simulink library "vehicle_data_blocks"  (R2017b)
settings: Solver=ode1  StartTime=0.0  StopTime=Inf  FixedStep=0.001  RelTol=1e-3  EnableMultiTasking=on
PostLoadFcn:
  | , if any(exist('dsrtsu_mdlpostloadfcn', 'file') == [2, 3, 6]), try dsrtsu_mdlpostloadfcn('Execute', bdroot); catch fprintf('Error in PostLoadFcn (dsrtsu_mdlpostloadfcn) for model "%s":\n %s\n', bdroot, lasterr); end, end,
libraries: rtican x11

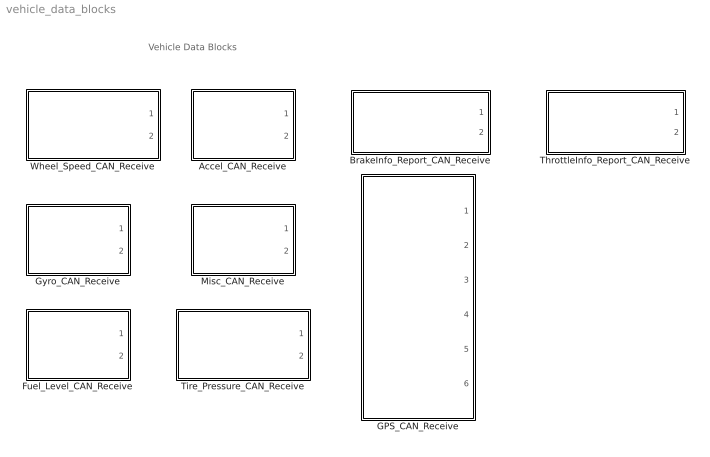
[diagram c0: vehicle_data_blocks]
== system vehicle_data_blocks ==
  note: Vehicle Data Blocks
  Accel_CAN_Receive : Subsystem
  BrakeInfo_Report_CAN_Receive : Subsystem
  Fuel_Level_CAN_Receive : Subsystem
  GPS_CAN_Receive : Subsystem
  Gyro_CAN_Receive : Subsystem
  Misc_CAN_Receive : Subsystem
  ThrottleInfo_Report_CAN_Receive : Subsystem
  Tire_Pressure_CAN_Receive : Subsystem
  Wheel_Speed_CAN_Receive : Subsystem

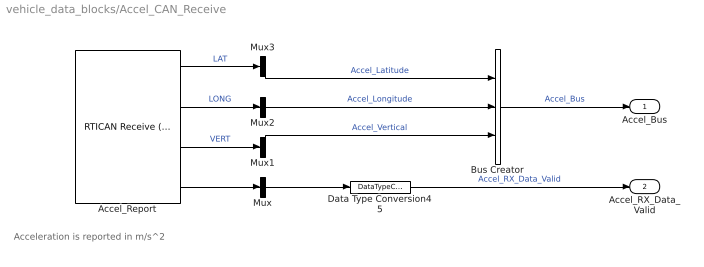
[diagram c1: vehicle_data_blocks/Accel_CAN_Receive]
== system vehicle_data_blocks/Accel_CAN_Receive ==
  note: Acceleration is reported in m/s^2
  Accel_Report : rtican/RTICAN Receive (RX)   Reserved1=[]  Reserved2=[]  Reserved3=[]  Reserved4=[]  SfcnMessage=[]  Msg_Struct=[]  BoardTypeNo=[]  BoardNo=[]  ChannelNo=[]  Parameters=[]  DialogFcn=[]  UnitName=[]  Revision=[]  UnitValues=[]  DSProperties=struct('RTI',struct('Version',uint32(5),'BlockType',struct('isSLSource',uint8(1),'isSLSink',uint8(1),'isHWSource',uint8(0),'isHWSink',uint8(0),'isSetup',uint8(0),'isInline',uint8(1),'isNonInline',uint8(0),'isInterrupt',uint8(0),'isChannelwise',uint8(0)),'IOBoardType','RTICAN','UnitType','MESSAGE','Identifier','RX','DialogType','MSVC','BlockSet','RTICAN','SlaveProcessor','CAN'))  RTIBlockInterface=struct('OutputPortsWidth',int32([1 1 1 1]),'OutputPortsActive',[1 1 1 1],'OutputPortsName',{{'LAT','LONG','VERT',['RX status']}},'OutputPortsDataType',{{'SS_DOUBLE','SS_DOUBLE','SS_DOUBLE','SS_DOUBLE'}},'OutputPortsLabel',{{'LAT','LONG','VERT',''}},'OutputPortsLabelMode','ON','InputPortsWidth',int32(0),'InputPortsActive',0,'DialogFcn','rtican_message_interface_gui','BlockDisplay',{{'','center'}},'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  RTIBlockParameters=struct('BoardTypeNo',{{1,'OFF',[]}},'BoardNo',{{1,'ON',[1 16]}},'ChannelNo',{{1,'ON',[1 2]}},'Parameters',{{struct('DataFileSupport',struct('DataFileSelectedMaster',1,'DataFileSelectedLocal',1,'DataFileName','c:\repos\forddrivebywire\dataspeedbywire.dbc|','DataFileDate',['06-Sep-2016 16:47:06'],'SelectedFile','dataspeedbywire_20160909.dbc','InterfaceFcn','rtican_dbc_file_parser'),'Options',struct(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  RTISFcnParameters=struct('SFcnRTICANMessage','struct','TLCFileName','char')  RTIBlockParaDefault=struct('BoardTypeNo',4302,'BoardNo',1,'ChannelNo',1,'Parameters',struct('DataFileSupport',struct('DataFileSelectedMaster',0,'DataFileSelectedLocal',0,'DataFileName','','DataFileDate','','SelectedFile',['<no file selected>']),'Options',struct('StatusSelected',1,'TimeSelected',1,'DeltaTimeSelected',1,'BytePortSelected',0,'MessageLengthSelected',0,'TriggerPort',struct('Selected',0,'TriggerType','risi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
  Bus Creator : BusCreator  Inputs=3
  Data Type Conversion45 : DataTypeConversion  OutDataTypeStr=boolean
  Mux{,1..3} (4 alike) : Mux  Inputs=1
  Accel_Bus : Outport
  Accel_RX_Data_Valid : Outport  Port=2
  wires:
  Data Type Conversion45/1 -> Accel_RX_Data_Valid/1  "Accel_RX_Data_Valid"
  Mux1/1 -> Bus Creator/3  "Accel_Vertical"
  Mux2/1 -> Bus Creator/2  "Accel_Longitude"
  Mux3/1 -> Bus Creator/1  "Accel_Latitude"
  Mux/1 -> Data Type Conversion45/1
  Accel_Report/4 -> Mux/1
  Accel_Report/3 -> Mux1/1  "VERT"
  Accel_Report/2 -> Mux2/1  "LONG"
  Accel_Report/1 -> Mux3/1  "LAT"
  Bus Creator/1 -> Accel_Bus/1  "Accel_Bus"

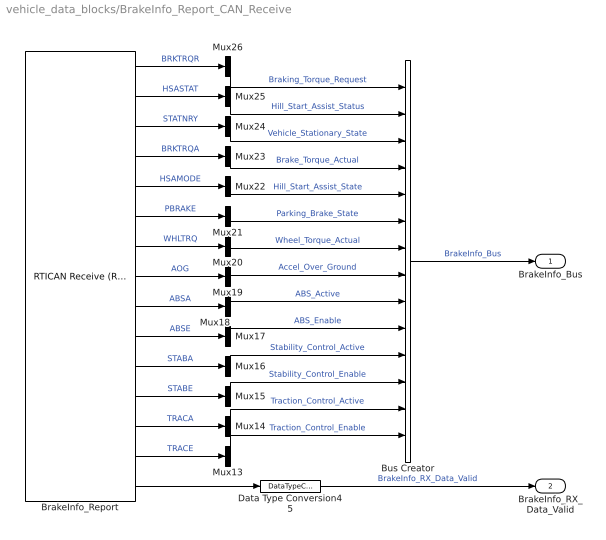
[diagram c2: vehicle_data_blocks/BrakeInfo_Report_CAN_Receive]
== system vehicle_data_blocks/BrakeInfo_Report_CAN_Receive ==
  BrakeInfo_Report : rtican/RTICAN Receive (RX)   Reserved1=[]  Reserved2=[]  Reserved3=[]  Reserved4=[]  SfcnMessage=[]  Msg_Struct=[]  BoardTypeNo=[]  BoardNo=[]  ChannelNo=[]  Parameters=[]  DialogFcn=[]  UnitName=[]  Revision=[]  UnitValues=[]  DSProperties=struct('RTI',struct('Version',uint32(5),'BlockType',struct('isSLSource',uint8(1),'isSLSink',uint8(1),'isHWSource',uint8(0),'isHWSink',uint8(0),'isSetup',uint8(0),'isInline',uint8(1),'isNonInline',uint8(0),'isInterrupt',uint8(0),'isChannelwise',uint8(0)),'IOBoardType','RTICAN','UnitType','MESSAGE','Identifier','RX','DialogType','MSVC','BlockSet','RTICAN','SlaveProcessor','CAN'))  RTIBlockInterface=struct('OutputPortsWidth',int32([1 1 1 1 1 1 1 1 1 1 1 1 1 1 1]),'OutputPortsActive',ones(1,15),'OutputPortsName',{{'BRKTRQR','HSASTAT','STATNRY','BRKTRQA','HSAMODE','PBRAKE','WHLTRQ','AOG','ABSA','ABSE','STABA','STABE','TRACA','TRACE',['RX status']}},'OutputPortsDataType',{{'SS_UINT16','SS_UINT8','SS_BOOLEAN','SS_UINT16','SS_UINT8','SS_UINT8','SS_INT16','SS_DOUBLE','SS_BOOLEAN','SS_BOOLEAN','SS_B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  RTIBlockParameters=struct('BoardTypeNo',{{1,'OFF',[]}},'BoardNo',{{1,'ON',[1 16]}},'ChannelNo',{{1,'ON',[1 2]}},'Parameters',{{struct('DataFileSupport',struct('DataFileSelectedMaster',1,'DataFileSelectedLocal',1,'DataFileName','c:\users\jsmith.dsi\documents\projects\forddrivebywire\dspace\lib\dataspeedbywire.dbc|','DataFileDate',['06-Sep-2016 16:47:06'],'SelectedFile','dataspeedbywire.dbc','InterfaceFcn','rtican_dbc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  RTISFcnParameters=struct('SFcnRTICANMessage','struct','TLCFileName','char')  RTIBlockParaDefault=struct('BoardTypeNo',4302,'BoardNo',1,'ChannelNo',1,'Parameters',struct('DataFileSupport',struct('DataFileSelectedMaster',0,'DataFileSelectedLocal',0,'DataFileName','','DataFileDate','','SelectedFile',['<no file selected>']),'Options',struct('StatusSelected',1,'TimeSelected',1,'DeltaTimeSelected',1,'BytePortSelected',0,'MessageLengthSelected',0,'TriggerPort',struct('Selected',0,'TriggerType','risi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
  Bus Creator : BusCreator  Inputs=14
  Data Type Conversion45 : DataTypeConversion  OutDataTypeStr=boolean
  Mux{13..26} (14 alike) : Mux  Inputs=1
  BrakeInfo_Bus : Outport
  BrakeInfo_RX_Data_Valid : Outport  Port=2
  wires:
  BrakeInfo_Report/15 -> Data Type Conversion45/1
  Data Type Conversion45/1 -> BrakeInfo_RX_Data_Valid/1  "BrakeInfo_RX_Data_Valid"
  BrakeInfo_Report/14 -> Mux13/1  "TRACE"
  BrakeInfo_Report/13 -> Mux14/1  "TRACA"
  BrakeInfo_Report/1 -> Mux26/1  "BRKTRQR"
  BrakeInfo_Report/2 -> Mux25/1  "HSASTAT"
  BrakeInfo_Report/3 -> Mux24/1  "STATNRY"
  BrakeInfo_Report/4 -> Mux23/1  "BRKTRQA"
  BrakeInfo_Report/5 -> Mux22/1  "HSAMODE"
  BrakeInfo_Report/6 -> Mux21/1  "PBRAKE"
  BrakeInfo_Report/7 -> Mux20/1  "WHLTRQ"
  BrakeInfo_Report/8 -> Mux19/1  "AOG"
  BrakeInfo_Report/9 -> Mux18/1  "ABSA"
  BrakeInfo_Report/10 -> Mux17/1  "ABSE"
  BrakeInfo_Report/11 -> Mux16/1  "STABA"
  BrakeInfo_Report/12 -> Mux15/1  "STABE"
  Mux20/1 -> Bus Creator/7  "Wheel_Torque_Actual"
  Mux15/1 -> Bus Creator/12  "Stability_Control_Enable"
  Mux18/1 -> Bus Creator/9  "ABS_Active"
  Mux16/1 -> Bus Creator/11  "Stability_Control_Active"
  Mux25/1 -> Bus Creator/2  "Hill_Start_Assist_Status"
  Mux26/1 -> Bus Creator/1  "Braking_Torque_Request"
  Mux17/1 -> Bus Creator/10  "ABS_Enable"
  Mux19/1 -> Bus Creator/8  "Accel_Over_Ground"
  Mux14/1 -> Bus Creator/13  "Traction_Control_Active"
  Mux24/1 -> Bus Creator/3  "Vehicle_Stationary_State"
  Mux22/1 -> Bus Creator/5  "Hill_Start_Assist_State"
  Mux13/1 -> Bus Creator/14  "Traction_Control_Enable"
  Mux21/1 -> Bus Creator/6  "Parking_Brake_State"
  Mux23/1 -> Bus Creator/4  "Brake_Torque_Actual"
  Bus Creator/1 -> BrakeInfo_Bus/1  "BrakeInfo_Bus"

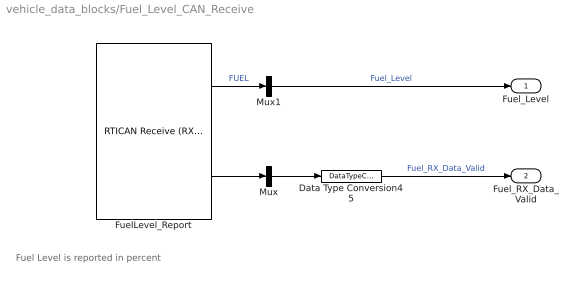
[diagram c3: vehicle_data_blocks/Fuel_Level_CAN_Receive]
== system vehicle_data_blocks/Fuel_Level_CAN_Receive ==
  note: Fuel Level is reported in percent
  Data Type Conversion45 : DataTypeConversion  OutDataTypeStr=boolean
  FuelLevel_Report : rtican/RTICAN Receive (RX)   Reserved1=[]  Reserved2=[]  Reserved3=[]  Reserved4=[]  SfcnMessage=[]  Msg_Struct=[]  BoardTypeNo=[]  BoardNo=[]  ChannelNo=[]  Parameters=[]  DialogFcn=[]  UnitName=[]  Revision=[]  UnitValues=[]  DSProperties=struct('RTI',struct('Version',uint32(5),'BlockType',struct('isSLSource',uint8(1),'isSLSink',uint8(1),'isHWSource',uint8(0),'isHWSink',uint8(0),'isSetup',uint8(0),'isInline',uint8(1),'isNonInline',uint8(0),'isInterrupt',uint8(0),'isChannelwise',uint8(0)),'IOBoardType','RTICAN','UnitType','MESSAGE','Identifier','RX','DialogType','MSVC','BlockSet','RTICAN','SlaveProcessor','CAN'))  RTIBlockInterface=struct('OutputPortsWidth',int32([1 1]),'OutputPortsActive',[1 1],'OutputPortsName',{{'FUEL',['RX status']}},'OutputPortsDataType',{{'SS_DOUBLE','SS_DOUBLE'}},'OutputPortsLabel',{{'FUEL',''}},'OutputPortsLabelMode','ON','InputPortsWidth',int32(0),'InputPortsActive',0,'DialogFcn','rtican_message_interface_gui','BlockDisplay',{{'','center'}},'IconTransparency','on','ParameterTunableNames',{{}},'InitL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  RTIBlockParameters=struct('BoardTypeNo',{{1,'OFF',[]}},'BoardNo',{{1,'ON',[1 16]}},'ChannelNo',{{1,'ON',[1 2]}},'Parameters',{{struct('DataFileSupport',struct('DataFileSelectedMaster',1,'DataFileSelectedLocal',1,'DataFileName','c:\repos\forddrivebywire\dataspeedbywire.dbc|','DataFileDate',['06-Sep-2016 16:47:06'],'SelectedFile','dataspeedbywire_20160909.dbc','InterfaceFcn','rtican_dbc_file_parser'),'Options',struct(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  RTISFcnParameters=struct('SFcnRTICANMessage','struct','TLCFileName','char')  RTIBlockParaDefault=struct('BoardTypeNo',4302,'BoardNo',1,'ChannelNo',1,'Parameters',struct('DataFileSupport',struct('DataFileSelectedMaster',0,'DataFileSelectedLocal',0,'DataFileName','','DataFileDate','','SelectedFile',['<no file selected>']),'Options',struct('StatusSelected',1,'TimeSelected',1,'DeltaTimeSelected',1,'BytePortSelected',0,'MessageLengthSelected',0,'TriggerPort',struct('Selected',0,'TriggerType','risi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
  Mux : Mux  Inputs=1
  Mux1 : Mux  Inputs=1
  Fuel_Level : Outport
  Fuel_RX_Data_Valid : Outport  Port=2
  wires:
  Data Type Conversion45/1 -> Fuel_RX_Data_Valid/1  "Fuel_RX_Data_Valid"
  Mux/1 -> Data Type Conversion45/1
  Mux1/1 -> Fuel_Level/1  "Fuel_Level"
  FuelLevel_Report/2 -> Mux/1
  FuelLevel_Report/1 -> Mux1/1  "FUEL"

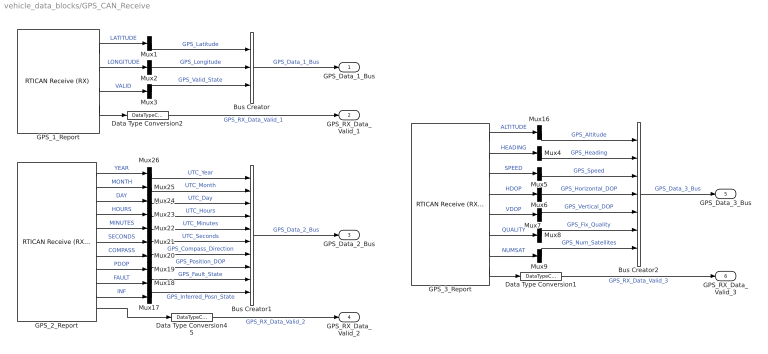
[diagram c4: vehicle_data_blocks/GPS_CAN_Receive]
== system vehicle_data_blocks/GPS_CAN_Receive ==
  Bus Creator : BusCreator  Inputs=3
  Bus Creator1 : BusCreator  Inputs=10
  Bus Creator2 : BusCreator  Inputs=7
  Data Type Conversion1 : DataTypeConversion  OutDataTypeStr=boolean
  Data Type Conversion2 : DataTypeConversion  OutDataTypeStr=boolean
  Data Type Conversion45 : DataTypeConversion  OutDataTypeStr=boolean
  GPS_1_Report : rtican/RTICAN Receive (RX)   Reserved1=[]  Reserved2=[]  Reserved3=[]  Reserved4=[]  SfcnMessage=[]  Msg_Struct=[]  BoardTypeNo=[]  BoardNo=[]  ChannelNo=[]  Parameters=[]  DialogFcn=[]  UnitName=[]  Revision=[]  UnitValues=[]  DSProperties=struct('RTI',struct('Version',uint32(5),'BlockType',struct('isSLSource',uint8(1),'isSLSink',uint8(1),'isHWSource',uint8(0),'isHWSink',uint8(0),'isSetup',uint8(0),'isInline',uint8(1),'isNonInline',uint8(0),'isInterrupt',uint8(0),'isChannelwise',uint8(0)),'IOBoardType','RTICAN','UnitType','MESSAGE','Identifier','RX','DialogType','MSVC','BlockSet','RTICAN','SlaveProcessor','CAN'))  RTIBlockInterface=struct('OutputPortsWidth',int32([1 1 1 1]),'OutputPortsActive',[1 1 1 1],'OutputPortsName',{{'LATITUDE','LONGITUDE','VALID',['RX status']}},'OutputPortsDataType',{{'SS_DOUBLE','SS_DOUBLE','SS_BOOLEAN','SS_DOUBLE'}},'OutputPortsLabel',{{'LATITUDE','LONGITUDE','VALID',''}},'OutputPortsLabelMode','ON','InputPortsWidth',int32(0),'InputPortsActive',0,'DialogFcn','rtican_message_interface_gui','BlockDis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  RTIBlockParameters=struct('BoardTypeNo',{{1,'OFF',[]}},'BoardNo',{{1,'ON',[1 16]}},'ChannelNo',{{1,'ON',[1 2]}},'Parameters',{{struct('DataFileSupport',struct('DataFileSelectedMaster',1,'DataFileSelectedLocal',1,'DataFileName','c:\repos\forddrivebywire\dataspeedbywire.dbc|','DataFileDate',{{{['16-Dec-2015 12:37:08']}}},'SelectedFile','..\..\..\..\dataspeedbywire.dbc'),'Options',struct('StatusSelected',1,'TimeSelecte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  RTISFcnParameters=struct('SFcnRTICANMessage','struct','TLCFileName','char')  RTIBlockParaDefault=struct('BoardTypeNo',4302,'BoardNo',1,'ChannelNo',1,'Parameters',struct('DataFileSupport',struct('DataFileSelectedMaster',0,'DataFileSelectedLocal',0,'DataFileName','','DataFileDate','','SelectedFile',['<no file selected>']),'Options',struct('StatusSelected',1,'TimeSelected',1,'DeltaTimeSelected',1,'BytePortSelected',0,'MessageLengthSelected',0,'TriggerPort',struct('Selected',0,'TriggerType','risi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
  GPS_2_Report : rtican/RTICAN Receive (RX)   Reserved1=[]  Reserved2=[]  Reserved3=[]  Reserved4=[]  SfcnMessage=[]  Msg_Struct=[]  BoardTypeNo=[]  BoardNo=[]  ChannelNo=[]  Parameters=[]  DialogFcn=[]  UnitName=[]  Revision=[]  UnitValues=[]  DSProperties=struct('RTI',struct('Version',uint32(5),'BlockType',struct('isSLSource',uint8(1),'isSLSink',uint8(1),'isHWSource',uint8(0),'isHWSink',uint8(0),'isSetup',uint8(0),'isInline',uint8(1),'isNonInline',uint8(0),'isInterrupt',uint8(0),'isChannelwise',uint8(0)),'IOBoardType','RTICAN','UnitType','MESSAGE','Identifier','RX','DialogType','MSVC','BlockSet','RTICAN','SlaveProcessor','CAN'))  RTIBlockInterface=struct('OutputPortsWidth',int32([1 1 1 1 1 1 1 1 1 1 1]),'OutputPortsActive',ones(1,11),'OutputPortsName',{{'YEAR','MONTH','DAY','HOURS','MINUTES','SECONDS','COMPASS','PDOP','FAULT','INF',['RX status']}},'OutputPortsDataType',{{'SS_UINT8','SS_UINT8','SS_UINT8','SS_UINT8','SS_UINT8','SS_UINT8','SS_UINT16','SS_DOUBLE','SS_BOOLEAN','SS_BOOLEAN','SS_DOUBLE'}},'OutputPortsLabel',{{'YEAR','MONTH','DAY',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  RTIBlockParameters=struct('BoardTypeNo',{{1,'OFF',[]}},'BoardNo',{{1,'ON',[1 16]}},'ChannelNo',{{1,'ON',[1 2]}},'Parameters',{{struct('DataFileSupport',struct('DataFileSelectedMaster',1,'DataFileSelectedLocal',1,'DataFileName','c:\repos\forddrivebywire\dataspeedbywire.dbc|','DataFileDate',{{{['16-Dec-2015 12:37:08']}}},'SelectedFile','..\..\..\..\dataspeedbywire.dbc'),'Options',struct('StatusSelected',1,'TimeSelecte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  RTISFcnParameters=struct('SFcnRTICANMessage','struct','TLCFileName','char')  RTIBlockParaDefault=struct('BoardTypeNo',4302,'BoardNo',1,'ChannelNo',1,'Parameters',struct('DataFileSupport',struct('DataFileSelectedMaster',0,'DataFileSelectedLocal',0,'DataFileName','','DataFileDate','','SelectedFile',['<no file selected>']),'Options',struct('StatusSelected',1,'TimeSelected',1,'DeltaTimeSelected',1,'BytePortSelected',0,'MessageLengthSelected',0,'TriggerPort',struct('Selected',0,'TriggerType','risi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
  GPS_3_Report : rtican/RTICAN Receive (RX)   Reserved1=[]  Reserved2=[]  Reserved3=[]  Reserved4=[]  SfcnMessage=[]  Msg_Struct=[]  BoardTypeNo=[]  BoardNo=[]  ChannelNo=[]  Parameters=[]  DialogFcn=[]  UnitName=[]  Revision=[]  UnitValues=[]  DSProperties=struct('RTI',struct('Version',uint32(5),'BlockType',struct('isSLSource',uint8(1),'isSLSink',uint8(1),'isHWSource',uint8(0),'isHWSink',uint8(0),'isSetup',uint8(0),'isInline',uint8(1),'isNonInline',uint8(0),'isInterrupt',uint8(0),'isChannelwise',uint8(0)),'IOBoardType','RTICAN','UnitType','MESSAGE','Identifier','RX','DialogType','MSVC','BlockSet','RTICAN','SlaveProcessor','CAN'))  RTIBlockInterface=struct('OutputPortsWidth',int32([1 1 1 1 1 1 1 1]),'OutputPortsActive',[1 1 1 1 1 1 1 1],'OutputPortsName',{{'ALTITUDE','HEADING','SPEED','HDOP','VDOP','QUALITY','NUMSAT',['RX status']}},'OutputPortsDataType',{{'SS_DOUBLE','SS_DOUBLE','SS_UINT8','SS_DOUBLE','SS_DOUBLE','SS_UINT8','SS_UINT8','SS_DOUBLE'}},'OutputPortsLabel',{{'ALTITUDE','HEADING','SPEED','HDOP','VDOP','QUALITY','NUMSAT',''}},'Outpu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  RTIBlockParameters=struct('BoardTypeNo',{{1,'OFF',[]}},'BoardNo',{{1,'ON',[1 16]}},'ChannelNo',{{1,'ON',[1 2]}},'Parameters',{{struct('DataFileSupport',struct('DataFileSelectedMaster',1,'DataFileSelectedLocal',1,'DataFileName','c:\repos\forddrivebywire\dataspeedbywire.dbc|','DataFileDate',{{{['16-Dec-2015 12:37:08']}}},'SelectedFile','..\..\..\..\dataspeedbywire.dbc'),'Options',struct('StatusSelected',1,'TimeSelecte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  RTISFcnParameters=struct('SFcnRTICANMessage','struct','TLCFileName','char')  RTIBlockParaDefault=struct('BoardTypeNo',4302,'BoardNo',1,'ChannelNo',1,'Parameters',struct('DataFileSupport',struct('DataFileSelectedMaster',0,'DataFileSelectedLocal',0,'DataFileName','','DataFileDate','','SelectedFile',['<no file selected>']),'Options',struct('StatusSelected',1,'TimeSelected',1,'DeltaTimeSelected',1,'BytePortSelected',0,'MessageLengthSelected',0,'TriggerPort',struct('Selected',0,'TriggerType','risi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
  Mux{1..9,16..26} (20 alike) : Mux  Inputs=1
  GPS_Data_1_Bus : Outport
  GPS_RX_Data_Valid_1 : Outport  Port=2
  GPS_Data_2_Bus : Outport  Port=3
  GPS_RX_Data_Valid_2 : Outport  Port=4
  GPS_Data_3_Bus : Outport  Port=5
  GPS_RX_Data_Valid_3 : Outport  Port=6
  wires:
  GPS_1_Report/1 -> Mux1/1  "LATITUDE"
  GPS_1_Report/2 -> Mux2/1  "LONGITUDE"
  GPS_1_Report/3 -> Mux3/1  "VALID"
  Bus Creator/1 -> GPS_Data_1_Bus/1  "GPS_Data_1_Bus"
  GPS_1_Report/4 -> Data Type Conversion2/1
  GPS_2_Report/1 -> Mux26/1  "YEAR"
  GPS_2_Report/2 -> Mux25/1  "MONTH"
  GPS_2_Report/3 -> Mux24/1  "DAY"
  GPS_2_Report/4 -> Mux23/1  "HOURS"
  GPS_2_Report/5 -> Mux22/1  "MINUTES"
  GPS_2_Report/6 -> Mux21/1  "SECONDS"
  GPS_2_Report/7 -> Mux20/1  "COMPASS"
  GPS_2_Report/8 -> Mux19/1  "PDOP"
  GPS_2_Report/9 -> Mux18/1  "FAULT"
  GPS_2_Report/10 -> Mux17/1  "INF"
  Bus Creator1/1 -> GPS_Data_2_Bus/1  "GPS_Data_2_Bus"
  GPS_2_Report/11 -> Data Type Conversion45/1
  GPS_3_Report/1 -> Mux16/1  "ALTITUDE"
  GPS_3_Report/2 -> Mux4/1  "HEADING"
  GPS_3_Report/3 -> Mux5/1  "SPEED"
  GPS_3_Report/4 -> Mux6/1  "HDOP"
  GPS_3_Report/5 -> Mux7/1  "VDOP"
  GPS_3_Report/6 -> Mux8/1  "QUALITY"
  GPS_3_Report/7 -> Mux9/1  "NUMSAT"
  Bus Creator2/1 -> GPS_Data_3_Bus/1  "GPS_Data_3_Bus"
  GPS_3_Report/8 -> Data Type Conversion1/1
  Data Type Conversion45/1 -> GPS_RX_Data_Valid_2/1  "GPS_RX_Data_Valid_2"
  Data Type Conversion1/1 -> GPS_RX_Data_Valid_3/1  "GPS_RX_Data_Valid_3"
  Data Type Conversion2/1 -> GPS_RX_Data_Valid_1/1  "GPS_RX_Data_Valid_1"
  Mux26/1 -> Bus Creator1/1  "UTC_Year"
  Mux25/1 -> Bus Creator1/2  "UTC_Month"
  Mux24/1 -> Bus Creator1/3  "UTC_Day"
  Mux23/1 -> Bus Creator1/4  "UTC_Hours"
  Mux22/1 -> Bus Creator1/5  "UTC_Minutes"
  Mux21/1 -> Bus Creator1/6  "UTC_Seconds"
  Mux20/1 -> Bus Creator1/7  "GPS_Compass_Direction"
  Mux19/1 -> Bus Creator1/8  "GPS_Position_DOP"
  Mux18/1 -> Bus Creator1/9  "GPS_Fault_State"
  Mux17/1 -> Bus Creator1/10  "GPS_Inferred_Posn_State"
  Mux1/1 -> Bus Creator/1  "GPS_Latitude"
  Mux2/1 -> Bus Creator/2  "GPS_Longitude"
  Mux3/1 -> Bus Creator/3  "GPS_Valid_State"
  Mux16/1 -> Bus Creator2/1  "GPS_Altitude"
  Mux4/1 -> Bus Creator2/2  "GPS_Heading"
  Mux5/1 -> Bus Creator2/3  "GPS_Speed"
  Mux6/1 -> Bus Creator2/4  "GPS_Horizontal_DOP"
  Mux7/1 -> Bus Creator2/5  "GPS_Vertical_DOP"
  Mux8/1 -> Bus Creator2/6  "GPS_Fix_Quality"
  Mux9/1 -> Bus Creator2/7  "GPS_Num_Satellites"

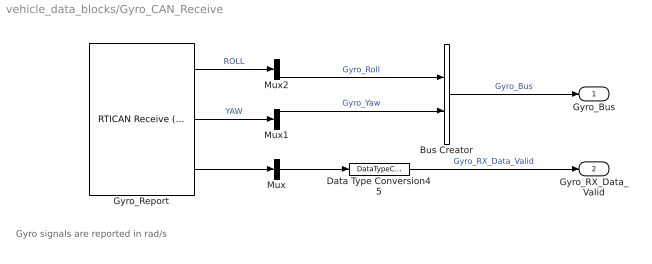
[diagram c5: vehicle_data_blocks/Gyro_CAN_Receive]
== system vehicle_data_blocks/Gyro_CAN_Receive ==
  note: Gyro signals are reported in rad/s
  Bus Creator : BusCreator  Inputs=2
  Data Type Conversion45 : DataTypeConversion  OutDataTypeStr=boolean
  Gyro_Report : rtican/RTICAN Receive (RX)   Reserved1=[]  Reserved2=[]  Reserved3=[]  Reserved4=[]  SfcnMessage=[]  Msg_Struct=[]  BoardTypeNo=[]  BoardNo=[]  ChannelNo=[]  Parameters=[]  DialogFcn=[]  UnitName=[]  Revision=[]  UnitValues=[]  DSProperties=struct('RTI',struct('Version',uint32(5),'BlockType',struct('isSLSource',uint8(1),'isSLSink',uint8(1),'isHWSource',uint8(0),'isHWSink',uint8(0),'isSetup',uint8(0),'isInline',uint8(1),'isNonInline',uint8(0),'isInterrupt',uint8(0),'isChannelwise',uint8(0)),'IOBoardType','RTICAN','UnitType','MESSAGE','Identifier','RX','DialogType','MSVC','BlockSet','RTICAN','SlaveProcessor','CAN'))  RTIBlockInterface=struct('OutputPortsWidth',int32([1 1 1]),'OutputPortsActive',[1 1 1],'OutputPortsName',{{'ROLL','YAW',['RX status']}},'OutputPortsDataType',{{'SS_DOUBLE','SS_DOUBLE','SS_DOUBLE'}},'OutputPortsLabel',{{'ROLL','YAW',''}},'OutputPortsLabelMode','ON','InputPortsWidth',int32(0),'InputPortsActive',0,'DialogFcn','rtican_message_interface_gui','BlockDisplay',{{'','center'}},'IconTransparency','on','Parame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  RTIBlockParameters=struct('BoardTypeNo',{{1,'OFF',[]}},'BoardNo',{{1,'ON',[1 16]}},'ChannelNo',{{1,'ON',[1 2]}},'Parameters',{{struct('DataFileSupport',struct('DataFileSelectedMaster',1,'DataFileSelectedLocal',1,'DataFileName','c:\repos\forddrivebywire\dataspeedbywire.dbc|','DataFileDate',['06-Sep-2016 16:47:06'],'SelectedFile','dataspeedbywire_20160909.dbc','InterfaceFcn','rtican_dbc_file_parser'),'Options',struct(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  RTISFcnParameters=struct('SFcnRTICANMessage','struct','TLCFileName','char')  RTIBlockParaDefault=struct('BoardTypeNo',4302,'BoardNo',1,'ChannelNo',1,'Parameters',struct('DataFileSupport',struct('DataFileSelectedMaster',0,'DataFileSelectedLocal',0,'DataFileName','','DataFileDate','','SelectedFile',['<no file selected>']),'Options',struct('StatusSelected',1,'TimeSelected',1,'DeltaTimeSelected',1,'BytePortSelected',0,'MessageLengthSelected',0,'TriggerPort',struct('Selected',0,'TriggerType','risi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
  Mux : Mux  Inputs=1
  Mux1 : Mux  Inputs=1
  Mux2 : Mux  Inputs=1
  Gyro_Bus : Outport
  Gyro_RX_Data_Valid : Outport  Port=2
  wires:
  Data Type Conversion45/1 -> Gyro_RX_Data_Valid/1  "Gyro_RX_Data_Valid"
  Mux1/1 -> Bus Creator/2  "Gyro_Yaw"
  Mux2/1 -> Bus Creator/1  "Gyro_Roll"
  Mux/1 -> Data Type Conversion45/1
  Gyro_Report/3 -> Mux/1
  Gyro_Report/2 -> Mux1/1  "YAW"
  Gyro_Report/1 -> Mux2/1  "ROLL"
  Bus Creator/1 -> Gyro_Bus/1  "Gyro_Bus"

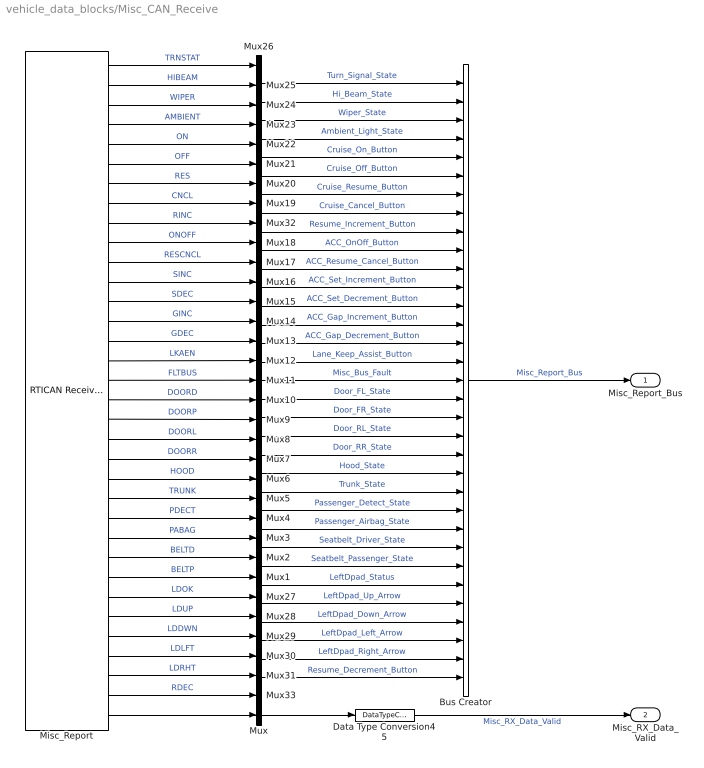
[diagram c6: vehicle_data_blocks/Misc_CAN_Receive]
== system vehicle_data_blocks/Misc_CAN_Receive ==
  Bus Creator : BusCreator  Inputs=33
  Data Type Conversion45 : DataTypeConversion  OutDataTypeStr=boolean
  Misc_Report : rtican/RTICAN Receive (RX)   Reserved1=[]  Reserved2=[]  Reserved3=[]  Reserved4=[]  SfcnMessage=[]  Msg_Struct=[]  BoardTypeNo=[]  BoardNo=[]  ChannelNo=[]  Parameters=[]  DialogFcn=[]  UnitName=[]  Revision=[]  UnitValues=[]  DSProperties=struct('RTI',struct('Version',uint32(5),'BlockType',struct('isSLSource',uint8(1),'isSLSink',uint8(1),'isHWSource',uint8(0),'isHWSink',uint8(0),'isSetup',uint8(0),'isInline',uint8(1),'isNonInline',uint8(0),'isInterrupt',uint8(0),'isChannelwise',uint8(0)),'IOBoardType','RTICAN','UnitType','MESSAGE','Identifier','RX','DialogType','MSVC','BlockSet','RTICAN','SlaveProcessor','CAN'))  RTIBlockInterface=struct('OutputPortsWidth',int32([1 1 1 1 1 1 1 1 1 1 1 1 1 1 1 1 1 1 1 1 1 1 1 1 1 1 1 1 1 1 1 1 1 1]),'OutputPortsActive',ones(1,34),'OutputPortsName',{{'TRNSTAT','HIBEAM','WIPER','AMBIENT','ON','OFF','RES','CNCL','RINC','ONOFF','RESCNCL','SINC','SDEC','GINC','GDEC','LKAEN','FLTBUS','DOORD','DOORP','DOORL','DOORR','HOOD','TRUNK','PDECT','PABAG','BELTD','BELTP','LDOK','LDUP','LDDWN','LDLFT','LDRHT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  RTIBlockParameters=struct('BoardTypeNo',{{1,'OFF',[]}},'BoardNo',{{1,'ON',[1 16]}},'ChannelNo',{{1,'ON',[1 2]}},'Parameters',{{struct('DataFileSupport',struct('DataFileSelectedMaster',1,'DataFileSelectedLocal',1,'DataFileName','c:\users\dataspeed\documents\projects\forddrivebywire\dspace\lib\dataspeedbywire.dbc|','DataFileDate',['06-Jun-2018 10:58:22'],'SelectedFile','dataspeedbywire.dbc','InterfaceFcn','rtican_dbc_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  RTISFcnParameters=struct('SFcnRTICANMessage','struct','TLCFileName','char')  RTIBlockParaDefault=struct('BoardTypeNo',4302,'BoardNo',1,'ChannelNo',1,'Parameters',struct('DataFileSupport',struct('DataFileSelectedMaster',0,'DataFileSelectedLocal',0,'DataFileName','','DataFileDate','','SelectedFile',['<no file selected>']),'Options',struct('StatusSelected',1,'TimeSelected',1,'DeltaTimeSelected',1,'BytePortSelected',0,'MessageLengthSelected',0,'TriggerPort',struct('Selected',0,'TriggerType','risi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
  Mux{,1..33} (34 alike) : Mux  Inputs=1
  Misc_Report_Bus : Outport
  Misc_RX_Data_Valid : Outport  Port=2
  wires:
  Misc_Report/32 -> Mux31/1  "LDRHT"
  Misc_Report/31 -> Mux30/1  "LDLFT"
  Misc_Report/30 -> Mux29/1  "LDDWN"
  Misc_Report/29 -> Mux28/1  "LDUP"
  Misc_Report/28 -> Mux27/1  "LDOK"
  Misc_Report/3 -> Mux24/1  "WIPER"
  Misc_Report/2 -> Mux25/1  "HIBEAM"
  Misc_Report/1 -> Mux26/1  "TRNSTAT"
  Mux23/1 -> Bus Creator/4  "Ambient_Light_State"
  Data Type Conversion45/1 -> Misc_RX_Data_Valid/1  "Misc_RX_Data_Valid"
  Mux19/1 -> Bus Creator/8  "Cruise_Cancel_Button"
  Mux20/1 -> Bus Creator/7  "Cruise_Resume_Button"
  Mux21/1 -> Bus Creator/6  "Cruise_Off_Button"
  Mux22/1 -> Bus Creator/5  "Cruise_On_Button"
  Mux24/1 -> Bus Creator/3  "Wiper_State"
  Mux25/1 -> Bus Creator/2  "Hi_Beam_State"
  Mux26/1 -> Bus Creator/1  "Turn_Signal_State"
  Mux/1 -> Data Type Conversion45/1
  Misc_Report/34 -> Mux/1
  Misc_Report/27 -> Mux1/1  "BELTP"
  Misc_Report/26 -> Mux2/1  "BELTD"
  Misc_Report/25 -> Mux3/1  "PABAG"
  Misc_Report/24 -> Mux4/1  "PDECT"
  Misc_Report/23 -> Mux5/1  "TRUNK"
  Misc_Report/22 -> Mux6/1  "HOOD"
  Misc_Report/21 -> Mux7/1  "DOORR"
  Misc_Report/20 -> Mux8/1  "DOORL"
  Misc_Report/19 -> Mux9/1  "DOORP"
  Misc_Report/18 -> Mux10/1  "DOORD"
  Misc_Report/17 -> Mux11/1  "FLTBUS"
  Misc_Report/16 -> Mux12/1  "LKAEN"
  Misc_Report/15 -> Mux13/1  "GDEC"
  Misc_Report/14 -> Mux14/1  "GINC"
  Misc_Report/13 -> Mux15/1  "SDEC"
  Misc_Report/12 -> Mux16/1  "SINC"
  Misc_Report/11 -> Mux17/1  "RESCNCL"
  Misc_Report/10 -> Mux18/1  "ONOFF"
  Misc_Report/8 -> Mux19/1  "CNCL"
  Misc_Report/7 -> Mux20/1  "RES"
  Misc_Report/6 -> Mux21/1  "OFF"
  Misc_Report/5 -> Mux22/1  "ON"
  Misc_Report/4 -> Mux23/1  "AMBIENT"
  Bus Creator/1 -> Misc_Report_Bus/1  "Misc_Report_Bus"
  Misc_Report/9 -> Mux32/1  "RINC"
  Misc_Report/33 -> Mux33/1  "RDEC"
  Mux32/1 -> Bus Creator/9  "Resume_Increment_Button"
  Mux18/1 -> Bus Creator/10  "ACC_OnOff_Button"
  Mux17/1 -> Bus Creator/11  "ACC_Resume_Cancel_Button"
  Mux16/1 -> Bus Creator/12  "ACC_Set_Increment_Button"
  Mux15/1 -> Bus Creator/13  "ACC_Set_Decrement_Button"
  Mux14/1 -> Bus Creator/14  "ACC_Gap_Increment_Button"
  Mux13/1 -> Bus Creator/15  "ACC_Gap_Decrement_Button"
  Mux12/1 -> Bus Creator/16  "Lane_Keep_Assist_Button"
  Mux11/1 -> Bus Creator/17  "Misc_Bus_Fault"
  Mux10/1 -> Bus Creator/18  "Door_FL_State"
  Mux9/1 -> Bus Creator/19  "Door_FR_State"
  Mux8/1 -> Bus Creator/20  "Door_RL_State"
  Mux7/1 -> Bus Creator/21  "Door_RR_State"
  Mux6/1 -> Bus Creator/22  "Hood_State"
  Mux5/1 -> Bus Creator/23  "Trunk_State"
  Mux4/1 -> Bus Creator/24  "Passenger_Detect_State"
  Mux3/1 -> Bus Creator/25  "Passenger_Airbag_State"
  Mux2/1 -> Bus Creator/26  "Seatbelt_Driver_State"
  Mux1/1 -> Bus Creator/27  "Seatbelt_Passenger_State"
  Mux27/1 -> Bus Creator/28  "LeftDpad_Status"
  Mux28/1 -> Bus Creator/29  "LeftDpad_Up_Arrow"
  Mux29/1 -> Bus Creator/30  "LeftDpad_Down_Arrow"
  Mux30/1 -> Bus Creator/31  "LeftDpad_Left_Arrow"
  Mux31/1 -> Bus Creator/32  "LeftDpad_Right_Arrow"
  Mux33/1 -> Bus Creator/33  "Resume_Decrement_Button"

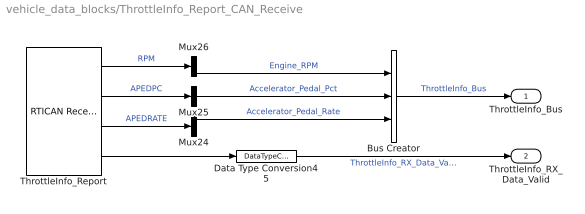
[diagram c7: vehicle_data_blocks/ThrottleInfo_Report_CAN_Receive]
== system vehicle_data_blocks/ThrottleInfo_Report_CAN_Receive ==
  Bus Creator : BusCreator  Inputs=3
  Data Type Conversion45 : DataTypeConversion  OutDataTypeStr=boolean
  Mux24 : Mux  Inputs=1
  Mux25 : Mux  Inputs=1
  Mux26 : Mux  Inputs=1
  ThrottleInfo_Report : rtican/RTICAN Receive (RX)   Reserved1=[]  Reserved2=[]  Reserved3=[]  Reserved4=[]  SfcnMessage=[]  Msg_Struct=[]  BoardTypeNo=[]  BoardNo=[]  ChannelNo=[]  Parameters=[]  DialogFcn=[]  UnitName=[]  Revision=[]  UnitValues=[]  DSProperties=struct('RTI',struct('Version',uint32(5),'BlockType',struct('isSLSource',uint8(1),'isSLSink',uint8(1),'isHWSource',uint8(0),'isHWSink',uint8(0),'isSetup',uint8(0),'isInline',uint8(1),'isNonInline',uint8(0),'isInterrupt',uint8(0),'isChannelwise',uint8(0)),'IOBoardType','RTICAN','UnitType','MESSAGE','Identifier','RX','DialogType','MSVC','BlockSet','RTICAN','SlaveProcessor','CAN'))  RTIBlockInterface=struct('OutputPortsWidth',int32([1 1 1 1]),'OutputPortsActive',[1 1 1 1],'OutputPortsName',{{'RPM','APEDPC','APEDRATE',['RX status']}},'OutputPortsDataType',{{'SS_DOUBLE','SS_DOUBLE','SS_DOUBLE','SS_DOUBLE'}},'OutputPortsLabel',{{'RPM','APEDPC','APEDRATE',''}},'OutputPortsLabelMode','ON','InputPortsWidth',int32(0),'InputPortsActive',0,'DialogFcn','rtican_message_interface_gui','BlockDisplay',{{'',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  RTIBlockParameters=struct('BoardTypeNo',{{1,'OFF',[]}},'BoardNo',{{1,'ON',[1 16]}},'ChannelNo',{{1,'ON',[1 2]}},'Parameters',{{struct('DataFileSupport',struct('DataFileSelectedMaster',1,'DataFileSelectedLocal',1,'DataFileName','c:\users\jsmith.dsi\documents\projects\forddrivebywire\dspace\lib\dataspeedbywire.dbc|','DataFileDate',{{{['11-Jul-2018 12:27:42']}}},'SelectedFile','dataspeedbywire.dbc','InterfaceFcn','rtic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  RTISFcnParameters=struct('SFcnRTICANMessage','struct','TLCFileName','char')  RTIBlockParaDefault=struct('BoardTypeNo',4302,'BoardNo',1,'ChannelNo',1,'Parameters',struct('DataFileSupport',struct('DataFileSelectedMaster',0,'DataFileSelectedLocal',0,'DataFileName','','DataFileDate','','SelectedFile',['<no file selected>']),'Options',struct('StatusSelected',1,'TimeSelected',1,'DeltaTimeSelected',1,'BytePortSelected',0,'MessageLengthSelected',0,'TriggerPort',struct('Selected',0,'TriggerType','risi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
  ThrottleInfo_Bus : Outport
  ThrottleInfo_RX_Data_Valid : Outport  Port=2
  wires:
  ThrottleInfo_Report/4 -> Data Type Conversion45/1
  Data Type Conversion45/1 -> ThrottleInfo_RX_Data_Valid/1  "ThrottleInfo_RX_Data_Valid"
  Mux25/1 -> Bus Creator/2  "Accelerator_Pedal_Pct"
  Mux26/1 -> Bus Creator/1  "Engine_RPM"
  Mux24/1 -> Bus Creator/3  "Accelerator_Pedal_Rate"
  Bus Creator/1 -> ThrottleInfo_Bus/1  "ThrottleInfo_Bus"
  ThrottleInfo_Report/1 -> Mux26/1  "RPM"
  ThrottleInfo_Report/2 -> Mux25/1  "APEDPC"
  ThrottleInfo_Report/3 -> Mux24/1  "APEDRATE"

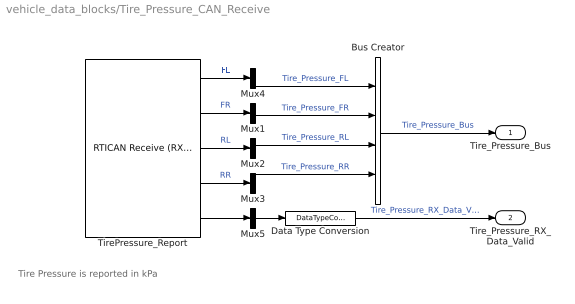
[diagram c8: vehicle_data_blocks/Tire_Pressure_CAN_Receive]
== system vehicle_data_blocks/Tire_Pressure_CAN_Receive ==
  note: Tire Pressure is reported in kPa
  Bus Creator : BusCreator  Inputs=4
  Data Type Conversion : DataTypeConversion  OutDataTypeStr=boolean
  Mux{1..5} (5 alike) : Mux  Inputs=1
  TirePressure_Report : rtican/RTICAN Receive (RX)   Reserved1=[]  Reserved2=[]  Reserved3=[]  Reserved4=[]  SfcnMessage=[]  Msg_Struct=[]  BoardTypeNo=[]  BoardNo=[]  ChannelNo=[]  Parameters=[]  DialogFcn=[]  UnitName=[]  Revision=[]  UnitValues=[]  DSProperties=struct('RTI',struct('Version',uint32(5),'BlockType',struct('isSLSource',uint8(1),'isSLSink',uint8(1),'isHWSource',uint8(0),'isHWSink',uint8(0),'isSetup',uint8(0),'isInline',uint8(1),'isNonInline',uint8(0),'isInterrupt',uint8(0),'isChannelwise',uint8(0)),'IOBoardType','RTICAN','UnitType','MESSAGE','Identifier','RX','DialogType','MSVC','BlockSet','RTICAN','SlaveProcessor','CAN'))  RTIBlockInterface=struct('OutputPortsWidth',int32([1 1 1 1 1]),'OutputPortsActive',[1 1 1 1 1],'OutputPortsName',{{'FL','FR','RL','RR',['RX status']}},'OutputPortsDataType',{{'SS_UINT16','SS_UINT16','SS_UINT16','SS_UINT16','SS_DOUBLE'}},'OutputPortsLabel',{{'FL','FR','RL','RR',''}},'OutputPortsLabelMode','ON','InputPortsWidth',int32(0),'InputPortsActive',0,'DialogFcn','rtican_message_interface_gui','BlockDisplay',{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  RTIBlockParameters=struct('BoardTypeNo',{{1,'OFF',[]}},'BoardNo',{{1,'ON',[1 16]}},'ChannelNo',{{1,'ON',[1 2]}},'Parameters',{{struct('DataFileSupport',struct('DataFileSelectedMaster',1,'DataFileSelectedLocal',1,'DataFileName','c:\repos\forddrivebywire\dataspeedbywire.dbc|','DataFileDate',{{{['16-Dec-2015 12:37:08']}}},'SelectedFile','..\..\..\..\dataspeedbywire.dbc'),'Options',struct('StatusSelected',1,'TimeSelecte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  RTISFcnParameters=struct('SFcnRTICANMessage','struct','TLCFileName','char')  RTIBlockParaDefault=struct('BoardTypeNo',4302,'BoardNo',1,'ChannelNo',1,'Parameters',struct('DataFileSupport',struct('DataFileSelectedMaster',0,'DataFileSelectedLocal',0,'DataFileName','','DataFileDate','','SelectedFile',['<no file selected>']),'Options',struct('StatusSelected',1,'TimeSelected',1,'DeltaTimeSelected',1,'BytePortSelected',0,'MessageLengthSelected',0,'TriggerPort',struct('Selected',0,'TriggerType','risi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
  Tire_Pressure_Bus : Outport
  Tire_Pressure_RX_Data_Valid : Outport  Port=2
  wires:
  TirePressure_Report/5 -> Mux5/1
  TirePressure_Report/1 -> Mux4/1  "FL"
  TirePressure_Report/2 -> Mux1/1  "FR"
  TirePressure_Report/3 -> Mux2/1  "RL"
  TirePressure_Report/4 -> Mux3/1  "RR"
  Bus Creator/1 -> Tire_Pressure_Bus/1  "Tire_Pressure_Bus"
  Mux4/1 -> Bus Creator/1  "Tire_Pressure_FL"
  Mux1/1 -> Bus Creator/2  "Tire_Pressure_FR"
  Mux2/1 -> Bus Creator/3  "Tire_Pressure_RL"
  Mux3/1 -> Bus Creator/4  "Tire_Pressure_RR"
  Mux5/1 -> Data Type Conversion/1
  Data Type Conversion/1 -> Tire_Pressure_RX_Data_Valid/1  "Tire_Pressure_RX_Data_Valid"

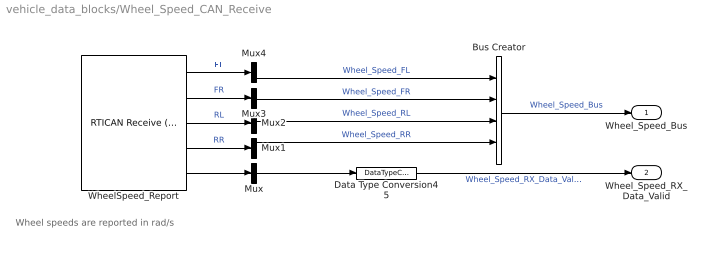
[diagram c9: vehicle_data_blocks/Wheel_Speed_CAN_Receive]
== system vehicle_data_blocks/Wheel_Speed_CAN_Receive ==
  note: Wheel speeds are reported in rad/s
  Bus Creator : BusCreator  Inputs=4
  Data Type Conversion45 : DataTypeConversion  OutDataTypeStr=boolean
  Mux{,1..4} (5 alike) : Mux  Inputs=1
  WheelSpeed_Report : rtican/RTICAN Receive (RX)   Reserved1=[]  Reserved2=[]  Reserved3=[]  Reserved4=[]  SfcnMessage=[]  Msg_Struct=[]  BoardTypeNo=[]  BoardNo=[]  ChannelNo=[]  Parameters=[]  DialogFcn=[]  UnitName=[]  Revision=[]  UnitValues=[]  DSProperties=struct('RTI',struct('Version',uint32(5),'BlockType',struct('isSLSource',uint8(1),'isSLSink',uint8(1),'isHWSource',uint8(0),'isHWSink',uint8(0),'isSetup',uint8(0),'isInline',uint8(1),'isNonInline',uint8(0),'isInterrupt',uint8(0),'isChannelwise',uint8(0)),'IOBoardType','RTICAN','UnitType','MESSAGE','Identifier','RX','DialogType','MSVC','BlockSet','RTICAN','SlaveProcessor','CAN'))  RTIBlockInterface=struct('OutputPortsWidth',int32([1 1 1 1 1]),'OutputPortsActive',[1 1 1 1 1],'OutputPortsName',{{'FL','FR','RL','RR',['RX status']}},'OutputPortsDataType',{{'SS_DOUBLE','SS_DOUBLE','SS_DOUBLE','SS_DOUBLE','SS_DOUBLE'}},'OutputPortsLabel',{{'FL','FR','RL','RR',''}},'OutputPortsLabelMode','ON','InputPortsWidth',int32(0),'InputPortsActive',0,'DialogFcn','rtican_message_interface_gui','BlockDisplay',{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  RTIBlockParameters=struct('BoardTypeNo',{{1,'OFF',[]}},'BoardNo',{{1,'ON',[1 16]}},'ChannelNo',{{1,'ON',[1 2]}},'Parameters',{{struct('DataFileSupport',struct('DataFileSelectedMaster',1,'DataFileSelectedLocal',1,'DataFileName','c:\repos\forddrivebywire\dataspeedbywire.dbc|','DataFileDate',['06-Sep-2016 16:47:06'],'SelectedFile','dataspeedbywire_20160909.dbc','InterfaceFcn','rtican_dbc_file_parser'),'Options',struct(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  RTISFcnParameters=struct('SFcnRTICANMessage','struct','TLCFileName','char')  RTIBlockParaDefault=struct('BoardTypeNo',4302,'BoardNo',1,'ChannelNo',1,'Parameters',struct('DataFileSupport',struct('DataFileSelectedMaster',0,'DataFileSelectedLocal',0,'DataFileName','','DataFileDate','','SelectedFile',['<no file selected>']),'Options',struct('StatusSelected',1,'TimeSelected',1,'DeltaTimeSelected',1,'BytePortSelected',0,'MessageLengthSelected',0,'TriggerPort',struct('Selected',0,'TriggerType','risi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
  Wheel_Speed_Bus : Outport
  Wheel_Speed_RX_Data_Valid : Outport  Port=2
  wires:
  Data Type Conversion45/1 -> Wheel_Speed_RX_Data_Valid/1  "Wheel_Speed_RX_Data_Valid"
  Mux1/1 -> Bus Creator/4  "Wheel_Speed_RR"
  Mux2/1 -> Bus Creator/3  "Wheel_Speed_RL"
  Mux3/1 -> Bus Creator/2  "Wheel_Speed_FR"
  Mux4/1 -> Bus Creator/1  "Wheel_Speed_FL"
  Mux/1 -> Data Type Conversion45/1
  WheelSpeed_Report/5 -> Mux/1
  WheelSpeed_Report/4 -> Mux1/1  "RR"
  WheelSpeed_Report/3 -> Mux2/1  "RL"
  WheelSpeed_Report/2 -> Mux3/1  "FR"
  WheelSpeed_Report/1 -> Mux4/1  "FL"
  Bus Creator/1 -> Wheel_Speed_Bus/1  "Wheel_Speed_Bus"
